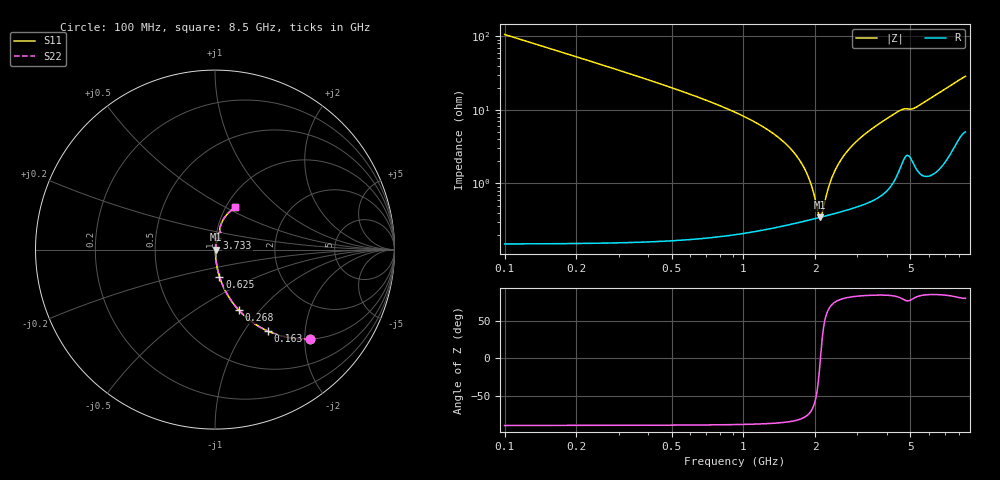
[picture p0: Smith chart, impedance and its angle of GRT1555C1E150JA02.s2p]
!Murata Part Number: GRT1555C1E150JA02
!These Parameters are Measured in Series Mode Connection
!Data Generated on Jun 19, 2026
!  o--ll--o
!Port1  Port2
!  o------o
!Operation Temp=25[degC], DC Bias Voltage=0[V]
!Freq. Start=100[MHz] Stop=9[GHz] 401[Steps]
# Hz S RI R 50
!Freq.(Hz) S11(Real) S11(Imag) S21(Real) S21(Imag) S12(Real) S12(Imag) S22(Real) S22(Imag)
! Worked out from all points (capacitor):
!   401 points, 100 MHz to 8.5 GHz, reference 50 ohm
!   read as one part in series: C = 15 pF near 142 MHz
!   lowest |Z| = 347 mohm at 2.095 GHz (marker M1)
!   series resonance near 2.101 GHz, so ESL is about 380 pH
!   S11 on the Smith chart (normalised r, x): 100 MHz: 1.00, -2.12; 163 MHz: 1.00, -1.29; 268 MHz: 1.00, -0.78; 625 MHz: 1.00, -0.31; 3.733 GHz: 1.01, +0.13; 8.5 GHz: 1.10, +0.56
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1e8  0.5284 -0.4985  0.4716 0.4985  0.4716 0.4985  0.5284 -0.4985
1.63e8  0.2955 -0.4551  0.7045 0.4551  0.7045 0.4551  0.2955 -0.4551
2.68e8  0.1327 -0.3373  0.8673 0.3373  0.8673 0.3373  0.1327 -0.3373
3.94e8  0.0645 -0.2427  0.9355 0.2427  0.9355 0.2427  0.0645 -0.2427
6.25e8  0.025 -0.1506  0.975 0.1506  0.975 0.1506  0.025 -0.1506
1.507e9  0.00384 -0.034  0.9962 0.034  0.9962 0.034  0.00384 -0.034
1.675e9  0.00343 -0.023  0.9966 0.023  0.9966 0.023  0.00343 -0.023
1.822e9  0.0033 -0.0144  0.9967 0.0144  0.9967 0.0144  0.0033 -0.0144
1.927e9  0.0033 -0.00874  0.9967 0.00874  0.9967 0.00874  0.0033 -0.00874
2.053e9  0.0034 -0.00234  0.9966 0.00234  0.9966 0.00234  0.0034 -0.00234
2.095e9  0.00345 -0.000288  0.9965 0.000288  0.9965 0.000288  0.00345 -0.000288
2.137e9  0.00351 0.00172  0.9965 -0.00172  0.9965 -0.00172  0.00351 0.00172
2.305e9  0.00383 0.00943  0.9962 -0.00943  0.9962 -0.00943  0.00383 0.00943
2.431e9  0.00414 0.0149  0.9959 -0.0149  0.9959 -0.0149  0.00414 0.0149
2.641e9  0.00477 0.0236  0.9952 -0.0236  0.9952 -0.0236  0.00477 0.0236
2.914e9  0.00582 0.0343  0.9942 -0.0343  0.9942 -0.0343  0.00582 0.0343
3.733e9  0.0108 0.0647  0.9892 -0.0647  0.9892 -0.0647  0.0108 0.0647
4.3e9  0.0185 0.0858  0.9815 -0.0858  0.9815 -0.0858  0.0185 0.0858
5.14e9  0.0283 0.0978  0.9717 -0.0978  0.9717 -0.0978  0.0283 0.0978
5.707e9  0.0275 0.1211  0.9725 -0.1211  0.9725 -0.1211  0.0275 0.1211
7.114e9  0.056 0.1827  0.944 -0.1827  0.944 -0.1827  0.056 0.1827
8.5e9  0.1114 0.2379  0.8886 -0.2379  0.8886 -0.2379  0.1114 0.2379
